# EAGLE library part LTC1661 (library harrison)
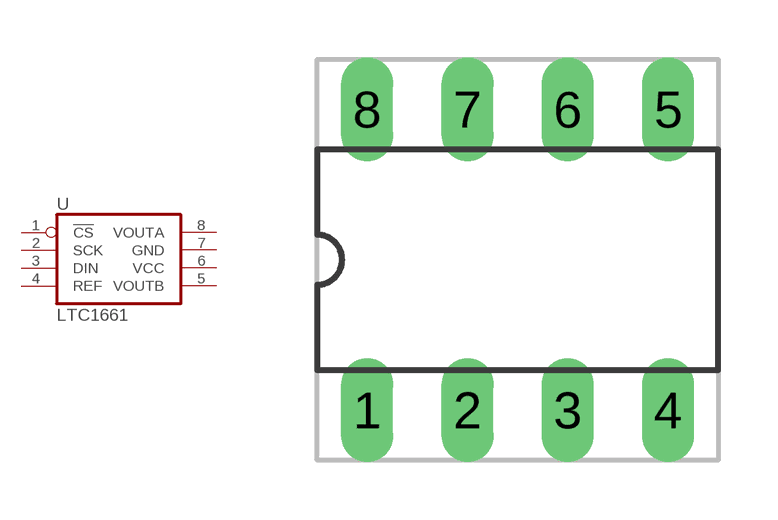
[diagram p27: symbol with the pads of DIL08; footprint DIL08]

Designator prefix U

## LTC1661  [DIL08]
1  !CS!  in
2  SCK  in
3  DIN  in
4  REF  in
5  VOUTB  out
6  VCC  pwr
7  GND  pwr
8  VOUTA  out

## Footprint DIL08 (pad centres in mm)
drill 0.813 long: 1 -3.81,-3.81; 2 -1.27,-3.81; 3 1.27,-3.81; 4 3.81,-3.81; 5 3.81,3.81; 6 1.27,3.81; 7 -1.27,3.81; 8 -3.81,3.81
